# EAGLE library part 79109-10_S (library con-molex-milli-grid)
RECEPTACAL
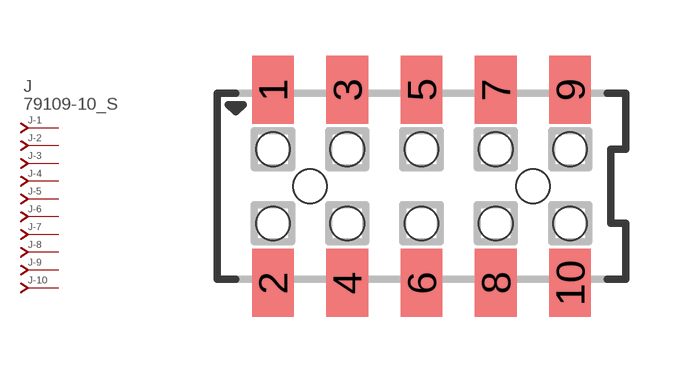
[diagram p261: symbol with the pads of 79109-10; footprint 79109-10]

Designator prefix J; gates -1=J-NV -2=J-N -3=J-N -4=J-N -5=J-N -6=J-N -7=J-N -8=J-N -9=J-N -10=J-N

## 79109-10_S  [79109-10]
1  -1:J  pas
2  -2:J  pas
3  -3:J  pas
4  -4:J  pas
5  -5:J  pas
6  -6:J  pas
7  -7:J  pas
8  -8:J  pas
9  -9:J  pas
10  -10:J  pas

## Footprint 79109-10 (pad centres in mm)
RECEPTACAL SMD Dual Row, Vertical, Pass-Thru
smd 1.12 x 1.83: 1 -4,2.6; 2 -4,-2.6; 3 -2,2.6; 4 -2,-2.6; 5 0,2.6; 6 0,-2.6; 7 2,2.6; 8 2,-2.6; 9 4,2.6; 10 4,-2.6
hole 0.914 at -3,0
hole 0.914 at -4,1
hole 0.914 at -4,-1
hole 0.914 at -2,-1
hole 0.914 at -2,1
hole 0.914 at 0,-1
hole 0.914 at 0,1
hole 0.914 at 3,0
hole 0.914 at 2,1
hole 0.914 at 2,-1
hole 0.914 at 4,1
hole 0.914 at 4,-1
